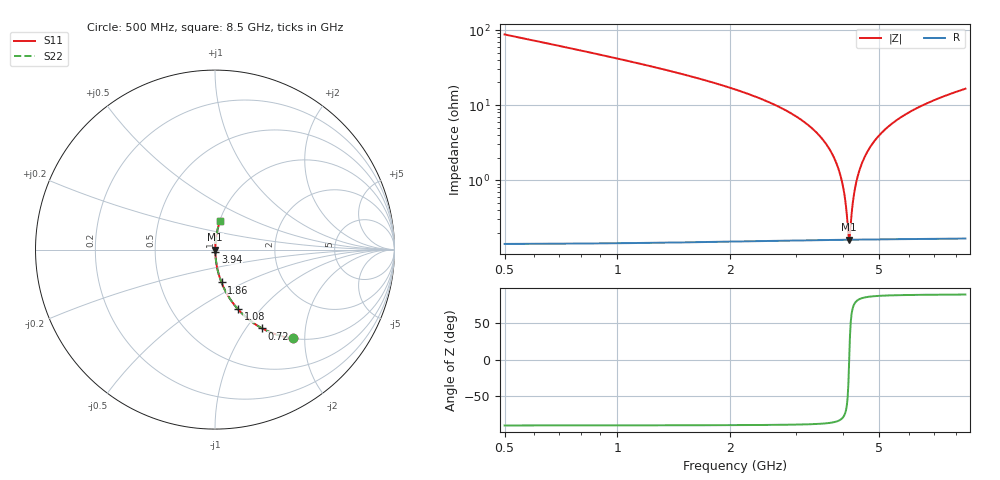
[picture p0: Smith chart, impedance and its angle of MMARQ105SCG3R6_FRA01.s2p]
! MMARQ105SCG3R6_FRA01  S-PARAMETER MODEL  ( General Type )
! Model Generated by TAIYO YUDEN Corporation (http://www.ty-top.com)
! Version 1.0
! TAIYO YUDEN Control No. 200326
! Copyright(c) 2020 TAIYO YUDEN CO.,LTD. All Rights Reserved.
! Product Description (link to TY-COMPAS)
! https://ds.yuden.co.jp/TYCOMPAS/or/detail?pn=MMARQ105SCG3R6BFRA01&u=M
! Products Name : Multilayer Ceramic Capacitors
! Characteristics :
!  Capacitance : 3.6 pF , Rated Voltage : 250V , TCC : CG / C0G
!  Case Size : 1.0 x 0.5 / 0.039 x 0.02 [mm/inch] , Thickness : 0.5 / 0.02 [mm/inch]
!  (Conditions: Temperature = 25 degC , DC Bias Current/Voltage = 0A / 0V)
! External Node Assignments :
!  1  o---| |---o  2
! GND o---------o GND
! Frequency Range : 500MHz  -  8.5GHz  [ 401 STEP ]
# MHz S RI R 50
! Freq[MHz].  S11 Real  S11 Imag  S21 Real  S21 Imag  S12 Real  S12 Imag  S22 Real  S22 Imag
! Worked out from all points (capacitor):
!   401 points, 500 MHz to 8.5 GHz, reference 50 ohm
!   read as one part in series: C = 3.6 pF near 540 MHz
!   lowest |Z| = 161 mohm at 4.16 GHz (marker M1)
!   series resonance near 4.16 GHz, so ESL is about 410 pH
!   S11 on the Smith chart (normalised r, x): 500 MHz: 1.00, -1.75; 720 MHz: 1.00, -1.19; 1.08 GHz: 1.00, -0.76; 1.86 GHz: 1.00, -0.38; 3.94 GHz: 1.00, -0.02; 8.5 GHz: 1.00, +0.33
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500  0.4323 -0.4946  0.5677 0.4946  0.5677 0.4946  0.4323 -0.4946
720  0.2628 -0.439  0.7372 0.439  0.7372 0.439  0.2628 -0.439
1080  0.1284 -0.3326  0.8716 0.3326  0.8716 0.3326  0.1284 -0.3326
1840  0.0374 -0.1859  0.9626 0.1859  0.9626 0.1859  0.0374 -0.1859
1860  0.0363 -0.1832  0.9637 0.1832  0.9637 0.1832  0.0363 -0.1832
3180  0.00489 -0.0575  0.9951 0.0575  0.9951 0.0575  0.00489 -0.0575
3660  0.00233 -0.0272  0.9977 0.0272  0.9977 0.0272  0.00233 -0.0272
3820  0.00192 -0.0181  0.9981 0.0181  0.9981 0.0181  0.00192 -0.0181
3940  0.00173 -0.0115  0.9983 0.0115  0.9983 0.0115  0.00173 -0.0115
4040  0.00164 -0.00621  0.9984 0.00621  0.9984 0.00621  0.00164 -0.00621
4120  0.00161 -0.00205  0.9984 0.00205  0.9984 0.00205  0.00161 -0.00205
4160  0.0016 -4.42e-06  0.9984 4.42e-06  0.9984 4.42e-06  0.0016 -4.42e-06
4200  0.00161 0.00202  0.9984 -0.00202  0.9984 -0.00202  0.00161 0.00202
4260  0.00163 0.00503  0.9984 -0.00503  0.9984 -0.00503  0.00163 0.00503
4320  0.00167 0.008  0.9983 -0.008  0.9983 -0.008  0.00167 0.008
4400  0.00175 0.0119  0.9982 -0.0119  0.9982 -0.0119  0.00175 0.0119
4500  0.00189 0.0167  0.9981 -0.0167  0.9981 -0.0167  0.00189 0.0167
4720  0.00234 0.0268  0.9977 -0.0268  0.9977 -0.0268  0.00234 0.0268
5000  0.00316 0.0391  0.9968 -0.0391  0.9968 -0.0391  0.00316 0.0391
5840  0.00698 0.0729  0.993 -0.0729  0.993 -0.0729  0.00698 0.0729
7180  0.0162 0.1197  0.9838 -0.1197  0.9838 -0.1197  0.0162 0.1197
8500  0.0281 0.1603  0.9719 -0.1603  0.9719 -0.1603  0.0281 0.1603
